DATA_BLOCK DB 50
TITLE =
VERSION : 1.0


 STRUCT
  OFFSET_TABLE: STRUCT
   Offset_Table : STRUCT
    Offset_Type : WORD := W#16#1;
    Offset_Length : WORD := W#16#1E;
    Offset_Address : WORD := W#16#0;
   END_STRUCT ;
   Processdata_Long_Table : STRUCT
    Processdata_Long_Type : WORD := W#16#6;
    Processdata_Long_Length : WORD := W#16#C;
    Processdata_Long_Address : WORD := W#16#1E;
   END_STRUCT ;
   Control_Table : STRUCT
    Control_Type : WORD := W#16#5;
    Control_Length : WORD := W#16#6;
    Control_Address : WORD := W#16#2A;
   END_STRUCT ;
   CAM_MT_Table : STRUCT
    CAM_MT_Type : WORD := W#16#7;
    CAM_MT_Length : WORD := W#16#3C;
    CAM_MT_Address : WORD := W#16#30;
   END_STRUCT ;
   Logic_Table : STRUCT
    Logic_Type : WORD := W#16#C;
    Logic_Length : WORD := W#16#5A;
    Logic_Address : WORD := W#16#6C;
   END_STRUCT ;
  END_STRUCT ;
  Processdata_Long_Table : STRUCT
   Position : DWORD := DW#16#0;
   Speed : WORD := W#16#0;
   Act_Prog : BYTE := B#16#0;
   ErrorNo : BYTE := B#16#0;
   Output1to8 : BYTE := B#16#0;
   Output9to16 : BYTE := B#16#0;
   Output17to24 : BYTE := B#16#0;
   Output25to32 : BYTE := B#16#0;
  END_STRUCT ;
  Control_Table : STRUCT
   New_Prog : BYTE := B#16#0;
   Teach_In_Zero : BOOL := FALSE;
   Invert_Encoder : BOOL := FALSE;
   Error_Quit : BOOL := FALSE;
   Res_03 : BOOL := FALSE;
   Res_04 : BOOL := FALSE;
   Res_05 : BOOL := FALSE;
   Res_06 : BOOL := FALSE;
   Res_07 : BOOL := FALSE;
   Res_0 : BYTE := B#16#0;
   Res_1 : BYTE := B#16#0;
   Res_2 : BYTE := B#16#0;
   Res_3 : BYTE := B#16#0;
  END_STRUCT ;
  CAM_MT_Table : STRUCT
   Cam_MT : ARRAY [ 1 .. 5 ] OF STRUCT
    ProgNo : WORD := W#16#0;
    Output : WORD := W#16#0;
    On : DWORD := DW#16#0;
    Off : DWORD := DW#16#0;
   END_STRUCT ;
  END_STRUCT ;
  Logic_Table : STRUCT
   Logic : ARRAY [ 1 .. 5 ] OF STRUCT
    ProgNo : BYTE := B#16#0;
    DestNo : BYTE := B#16#0;
    DestType : BYTE := B#16#0;
    OpNo1 : BYTE := B#16#0;
    OpType1 : BYTE := B#16#0;
    LogicFct1_2 : BYTE := B#16#0;
    OpNo2 : BYTE := B#16#0;
    OpType2 : BYTE := B#16#0;
    LogicFct2_3 : BYTE := B#16#0;
    OpNo3 : BYTE := B#16#0;
    OpType3 : BYTE := B#16#0;
    LogicFct3_4 : BYTE := B#16#0;
    OpNo4 : BYTE := B#16#0;
    OpType4 : BYTE := B#16#0;
    OutputDelay : WORD := W#16#0;
    OutputTrigger : BYTE := B#16#0;
    Modul_No : BYTE := B#16#0;
   END_STRUCT ;
  END_STRUCT ;
 END_STRUCT ;
BEGIN
   Offset_Table.Offset_Table.Offset_Type := W#16#1;
   Offset_Table.Offset_Table.Offset_Length := W#16#1E;
   Offset_Table.Offset_Table.Offset_Address := W#16#0;
   Offset_Table.Processdata_Long_Table.Processdata_Long_Type := W#16#6;
   Offset_Table.Processdata_Long_Table.Processdata_Long_Length := W#16#C;
   Offset_Table.Processdata_Long_Table.Processdata_Long_Address := W#16#1E;
   Offset_Table.Control_Table.Control_Type := W#16#5;
   Offset_Table.Control_Table.Control_Length := W#16#6;
   Offset_Table.Control_Table.Control_Address := W#16#2A;
   Offset_Table.CAM_MT_Table.CAM_MT_Type := W#16#7;
   Offset_Table.CAM_MT_Table.CAM_MT_Length := W#16#3C;
   Offset_Table.CAM_MT_Table.CAM_MT_Address := W#16#30;
   Offset_Table.Logic_Table.Logic_Type := W#16#C;
   Offset_Table.Logic_Table.Logic_Length := W#16#5A;
   Offset_Table.Logic_Table.Logic_Address := W#16#6C;
   Processdata_Long_Table.Position := DW#16#0;
   Processdata_Long_Table.Speed := W#16#0;
   Processdata_Long_Table.Act_Prog := B#16#0;
   Processdata_Long_Table.ErrorNo := B#16#0;
   Processdata_Long_Table.Output1to8 := B#16#0;
   Processdata_Long_Table.Output9to16 := B#16#0;
   Processdata_Long_Table.Output17to24 := B#16#0;
   Processdata_Long_Table.Output25to32 := B#16#0;
   Control_Table.New_Prog := B#16#0;
   Control_Table.Teach_In_Zero := FALSE;
   Control_Table.Invert_Encoder := FALSE;
   Control_Table.Error_Quit := FALSE;
   Control_Table.Res_03 := FALSE;
   Control_Table.Res_04 := FALSE;
   Control_Table.Res_05 := FALSE;
   Control_Table.Res_06 := FALSE;
   Control_Table.Res_07 := FALSE;
   Control_Table.Res_0 := B#16#0;
   Control_Table.Res_1 := B#16#0;
   Control_Table.Res_2 := B#16#0;
   Control_Table.Res_3 := B#16#0;
   CAM_MT_Table.Cam_MT[1].ProgNo := W#16#0;
   CAM_MT_Table.Cam_MT[1].Output := W#16#0;
   CAM_MT_Table.Cam_MT[1].On := DW#16#0;
   CAM_MT_Table.Cam_MT[1].Off := DW#16#0;
   CAM_MT_Table.Cam_MT[2].ProgNo := W#16#0;
   CAM_MT_Table.Cam_MT[2].Output := W#16#0;
   CAM_MT_Table.Cam_MT[2].On := DW#16#0;
   CAM_MT_Table.Cam_MT[2].Off := DW#16#0;
   CAM_MT_Table.Cam_MT[3].ProgNo := W#16#0;
   CAM_MT_Table.Cam_MT[3].Output := W#16#0;
   CAM_MT_Table.Cam_MT[3].On := DW#16#0;
   CAM_MT_Table.Cam_MT[3].Off := DW#16#0;
   CAM_MT_Table.Cam_MT[4].ProgNo := W#16#0;
   CAM_MT_Table.Cam_MT[4].Output := W#16#0;
   CAM_MT_Table.Cam_MT[4].On := DW#16#0;
   CAM_MT_Table.Cam_MT[4].Off := DW#16#0;
   CAM_MT_Table.Cam_MT[5].ProgNo := W#16#0;
   CAM_MT_Table.Cam_MT[5].Output := W#16#0;
   CAM_MT_Table.Cam_MT[5].On := DW#16#0;
   CAM_MT_Table.Cam_MT[5].Off := DW#16#0;
   Logic_Table.Logic[1].ProgNo := B#16#0;
   Logic_Table.Logic[1].DestNo := B#16#0;
   Logic_Table.Logic[1].DestType := B#16#0;
   Logic_Table.Logic[1].OpNo1 := B#16#0;
   Logic_Table.Logic[1].OpType1 := B#16#0;
   Logic_Table.Logic[1].LogicFct1_2 := B#16#0;
   Logic_Table.Logic[1].OpNo2 := B#16#0;
   Logic_Table.Logic[1].OpType2 := B#16#0;
   Logic_Table.Logic[1].LogicFct2_3 := B#16#0;
   Logic_Table.Logic[1].OpNo3 := B#16#0;
   Logic_Table.Logic[1].OpType3 := B#16#0;
   Logic_Table.Logic[1].LogicFct3_4 := B#16#0;
   Logic_Table.Logic[1].OpNo4 := B#16#0;
   Logic_Table.Logic[1].OpType4 := B#16#0;
   Logic_Table.Logic[1].OutputDelay := W#16#0;
   Logic_Table.Logic[1].OutputTrigger := B#16#0;
   Logic_Table.Logic[1].Modul_No := B#16#0;
   Logic_Table.Logic[2].ProgNo := B#16#0;
   Logic_Table.Logic[2].DestNo := B#16#0;
   Logic_Table.Logic[2].DestType := B#16#0;
   Logic_Table.Logic[2].OpNo1 := B#16#0;
   Logic_Table.Logic[2].OpType1 := B#16#0;
   Logic_Table.Logic[2].LogicFct1_2 := B#16#0;
   Logic_Table.Logic[2].OpNo2 := B#16#0;
   Logic_Table.Logic[2].OpType2 := B#16#0;
   Logic_Table.Logic[2].LogicFct2_3 := B#16#0;
   Logic_Table.Logic[2].OpNo3 := B#16#0;
   Logic_Table.Logic[2].OpType3 := B#16#0;
   Logic_Table.Logic[2].LogicFct3_4 := B#16#0;
   Logic_Table.Logic[2].OpNo4 := B#16#0;
   Logic_Table.Logic[2].OpType4 := B#16#0;
   Logic_Table.Logic[2].OutputDelay := W#16#0;
   Logic_Table.Logic[2].OutputTrigger := B#16#0;
   Logic_Table.Logic[2].Modul_No := B#16#0;
   Logic_Table.Logic[3].ProgNo := B#16#0;
   Logic_Table.Logic[3].DestNo := B#16#0;
   Logic_Table.Logic[3].DestType := B#16#0;
   Logic_Table.Logic[3].OpNo1 := B#16#0;
   Logic_Table.Logic[3].OpType1 := B#16#0;
   Logic_Table.Logic[3].LogicFct1_2 := B#16#0;
   Logic_Table.Logic[3].OpNo2 := B#16#0;
   Logic_Table.Logic[3].OpType2 := B#16#0;
   Logic_Table.Logic[3].LogicFct2_3 := B#16#0;
   Logic_Table.Logic[3].OpNo3 := B#16#0;
   Logic_Table.Logic[3].OpType3 := B#16#0;
   Logic_Table.Logic[3].LogicFct3_4 := B#16#0;
   Logic_Table.Logic[3].OpNo4 := B#16#0;
   Logic_Table.Logic[3].OpType4 := B#16#0;
   Logic_Table.Logic[3].OutputDelay := W#16#0;
   Logic_Table.Logic[3].OutputTrigger := B#16#0;
   Logic_Table.Logic[3].Modul_No := B#16#0;
   Logic_Table.Logic[4].ProgNo := B#16#0;
   Logic_Table.Logic[4].DestNo := B#16#0;
   Logic_Table.Logic[4].DestType := B#16#0;
   Logic_Table.Logic[4].OpNo1 := B#16#0;
   Logic_Table.Logic[4].OpType1 := B#16#0;
   Logic_Table.Logic[4].LogicFct1_2 := B#16#0;
   Logic_Table.Logic[4].OpNo2 := B#16#0;
   Logic_Table.Logic[4].OpType2 := B#16#0;
   Logic_Table.Logic[4].LogicFct2_3 := B#16#0;
   Logic_Table.Logic[4].OpNo3 := B#16#0;
   Logic_Table.Logic[4].OpType3 := B#16#0;
   Logic_Table.Logic[4].LogicFct3_4 := B#16#0;
   Logic_Table.Logic[4].OpNo4 := B#16#0;
   Logic_Table.Logic[4].OpType4 := B#16#0;
   Logic_Table.Logic[4].OutputDelay := W#16#0;
   Logic_Table.Logic[4].OutputTrigger := B#16#0;
   Logic_Table.Logic[4].Modul_No := B#16#0;
   Logic_Table.Logic[5].ProgNo := B#16#0;
   Logic_Table.Logic[5].DestNo := B#16#0;
   Logic_Table.Logic[5].DestType := B#16#0;
   Logic_Table.Logic[5].OpNo1 := B#16#0;
   Logic_Table.Logic[5].OpType1 := B#16#0;
   Logic_Table.Logic[5].LogicFct1_2 := B#16#0;
   Logic_Table.Logic[5].OpNo2 := B#16#0;
   Logic_Table.Logic[5].OpType2 := B#16#0;
   Logic_Table.Logic[5].LogicFct2_3 := B#16#0;
   Logic_Table.Logic[5].OpNo3 := B#16#0;
   Logic_Table.Logic[5].OpType3 := B#16#0;
   Logic_Table.Logic[5].LogicFct3_4 := B#16#0;
   Logic_Table.Logic[5].OpNo4 := B#16#0;
   Logic_Table.Logic[5].OpType4 := B#16#0;
   Logic_Table.Logic[5].OutputDelay := W#16#0;
   Logic_Table.Logic[5].OutputTrigger := B#16#0;
   Logic_Table.Logic[5].Modul_No := B#16#0;
END_DATA_BLOCK
